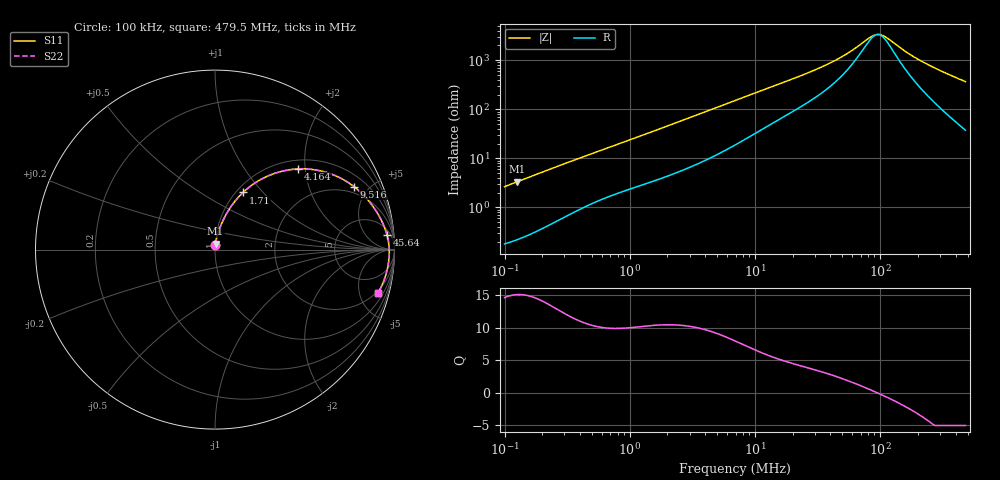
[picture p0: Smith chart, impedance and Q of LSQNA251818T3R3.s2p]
! LSQNA251818T3R3  S-PARAMETER MODEL  ( General Type )
! Model Generated by TAIYO YUDEN Corporation (http://www.ty-top.com)
! Version 2.0
! TAIYO YUDEN Control No. 100810NF25SB-FKC
! Copyright(c) 2007 TAIYO YUDEN CO.,LTD. All Rights Reserved.
! Product Description (link to TY-COMPAS)
! https://ds.yuden.co.jp/TYCOMPAS/or/detail?pn=LSQNA251818T3R3M&u=M
! Products Name : Inductors
! Characteristics :
!  Inductance : 3.3 uH , SRF(min) : 54 MHz , DC Resistance(max) : 0.143 Ohm
!  Rated Current : Saturation :440 mA , Temp Rise : 1200 mA (40 degC)
!  Case Size : 2.5 x 1.8 / 0.098 x 0.071 [mm/inch] , Thickness : 1.8 / 0.071 [mm/inch]
!  (Conditions: Temperature = 25 degC , DC Bias Current/Voltage = 0A / 0V)
! External Node Assignments :
!  1  o---GGG---o  2
! GND o---------o GND
! Frequency Range : 0.1MHz  -  479.524407MHz  [ 402 STEP ]
# MHz S RI R 50
! Freq[MHz].  S11 Real  S11 Imag  S21 Real  S21 Imag  S12 Real  S12 Imag  S22 Real  S22 Imag
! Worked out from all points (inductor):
!   401 points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, 100 kHz to 479.5 MHz, reference 50 ohm
!   read as one part in series: L = 4.2 uH near 104.3 kHz
!   highest Q = 15.1 at 126.2 kHz (marker M1), where L = 4.2 uH
!   self-resonance near 95.44 MHz
!   S11 on the Smith chart (normalised r, x): 100 kHz: 1.00, +0.05; 1.71 MHz: 1.08, +0.78; 4.164 MHz: 1.19, +1.84; 9.516 MHz: 1.59, +4.04; 45.64 MHz: 9, +19; 479.5 MHz: 1.75, -7.28
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0.1  0.0025 0.0264  0.9975 -0.0264  0.9975 -0.0264  0.0025 0.0264
0.126247  0.0033 0.0331  0.9967 -0.0331  0.9967 -0.0331  0.0033 0.0331
0.413557  0.02 0.1014  0.98 -0.1014  0.98 -0.1014  0.02 0.1014
0.944963  0.0669 0.2047  0.9331 -0.2047  0.9331 -0.2047  0.0669 0.2047
1.710297  0.1565 0.3187  0.8435 -0.3187  0.8435 -0.3187  0.1565 0.3187
2.612836  0.2767 0.4019  0.7233 -0.4019  0.7233 -0.4019  0.2767 0.4019
4.164441  0.4635 0.4495  0.5365 -0.4495  0.5365 -0.4495  0.4635 0.4495
5.370083  0.5733 0.4416  0.4267 -0.4416  0.4267 -0.4416  0.5733 0.4416
7.073061  0.6816 0.407  0.3184 -0.407  0.3184 -0.407  0.6816 0.407
9.515591  0.7748 0.3506  0.2252 -0.3506  0.2252 -0.3506  0.7748 0.3506
15.4911  0.8736 0.2497  0.1264 -0.2497  0.1264 -0.2497  0.8736 0.2497
28.6379  0.9358 0.1442  0.0642 -0.1442  0.0642 -0.1442  0.9358 0.1442
45.64422  0.9585 0.0816  0.0415 -0.0816  0.0415 -0.0816  0.9585 0.0816
57.62461  0.9648 0.0543  0.0352 -0.0543  0.0352 -0.0543  0.9648 0.0543
80.87987  0.9699 0.0174  0.0301 -0.0174  0.0301 -0.0174  0.9699 0.0174
89.91882  0.9707 0.00628  0.0293 -0.00628  0.0293 -0.00628  0.9707 0.00628
102.1087  0.9711 -0.00714  0.0289 0.00714  0.0289 0.00714  0.9711 -0.00714
118.4342  0.9711 -0.023  0.0289 0.023  0.0289 0.023  0.9711 -0.023
159.3329  0.9689 -0.0567  0.0311 0.0567  0.0311 0.0567  0.9689 -0.0567
214.355  0.9632 -0.0949  0.0368 0.0949  0.0368 0.0949  0.9632 -0.0949
320.6064  0.9461 -0.1587  0.0539 0.1587  0.0539 0.1587  0.9461 -0.1587
479.5244  0.9092 -0.2405  0.0908 0.2405  0.0908 0.2405  0.9092 -0.2405
